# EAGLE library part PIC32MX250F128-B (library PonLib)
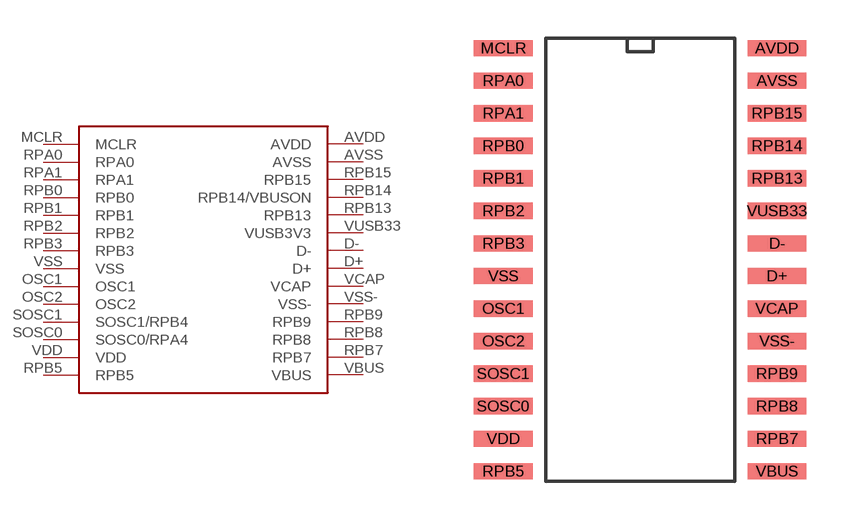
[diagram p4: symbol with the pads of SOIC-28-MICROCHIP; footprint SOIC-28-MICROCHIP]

Designator prefix -

## PIC32MX250F128-B  [SOIC-28-MICROCHIP]
AVDD  AVDD
AVSS  AVSS
D+  D+
D-  D-
MCLR  MCLR
OSC1  OSC1
OSC2  OSC2
RPA0  RPA0
RPA1  RPA1
RPB0  RPB0
RPB1  RPB1
RPB2  RPB2
RPB3  RPB3
RPB5  RPB5
RPB7  RPB7
RPB8  RPB8
RPB9  RPB9
RPB13  RPB13
RPB14  RPB14/VBUSON
RPB15  RPB15
SOSC0  SOSC0/RPA4
SOSC1  SOSC1/RPB4
VBUS  VBUS
VCAP  VCAP
VDD  VDD
VSS  VSS
VSS-  VSS-
VUSB33  VUSB3V3

## Footprint SOIC-28-MICROCHIP (pad centres in mm)
smd 2.286 x 0.635: AVDD 5.334,8.255; AVSS 5.334,6.985; D+ 5.334,-0.635; D- 5.334,0.635; MCLR -5.334,8.255; OSC1 -5.334,-1.905; OSC2 -5.334,-3.175; RPA0 -5.334,6.985; RPA1 -5.334,5.715; RPB0 -5.334,4.445; RPB1 -5.334,3.175; RPB2 -5.334,1.905; RPB3 -5.334,0.635; RPB5 -5.334,-8.255; RPB7 5.334,-6.985; RPB8 5.334,-5.715; RPB9 5.334,-4.445; RPB13 5.334,3.175; RPB14 5.334,4.445; RPB15 5.334,5.715; SOSC0 -5.334,-5.715; SOSC1 -5.334,-4.445; VBUS 5.334,-8.255; VCAP 5.334,-1.905; VDD -5.334,-6.985; VSS -5.334,-0.635; VSS- 5.334,-3.175; VUSB33 5.334,1.905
